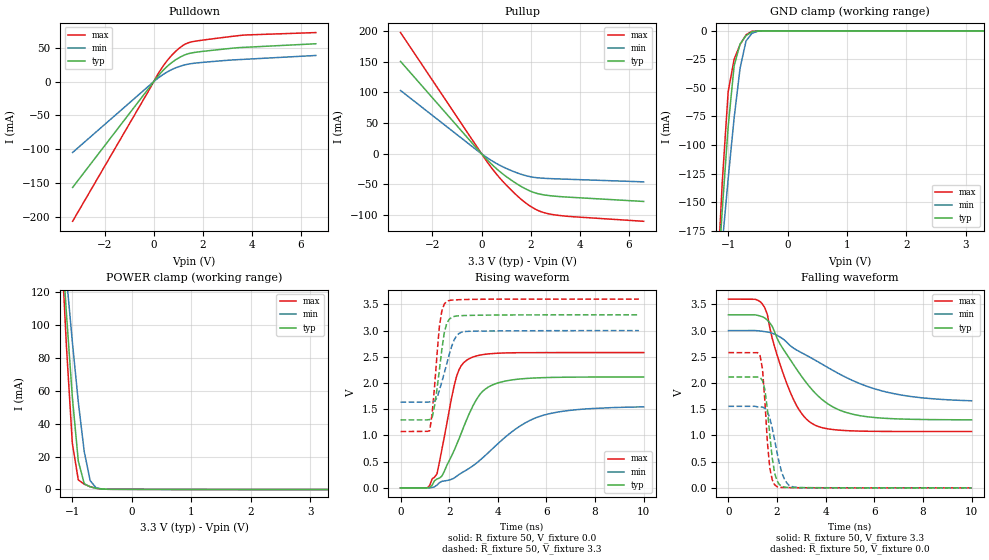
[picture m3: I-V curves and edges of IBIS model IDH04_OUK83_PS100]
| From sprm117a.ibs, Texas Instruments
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[Model]   IDH04_OUK83_PS100
| I/O with pullup
Model_type   I/O
Vinh = 2.00
Vinl = 0.80
Enable   Active-Low
Polarity   Non-Inverting
| signals   A, GZ, Y
Vmeas = 1.5
|   typ   min   max
C_comp   2.866p   2.862p   2.867p
|   typ   min   max
[Temperature Range]   25   -40   125
|   typ   min   max
[Voltage Range]   3.30V   3.00V   3.60V
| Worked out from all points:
|   slope of the pulldown table from 0 to 0.495 V, typ, clamps not added: 23.8 ohm
|   slope of the pullup table from 0 to 0.495 V, typ, clamps not added: 24.4 ohm
|   GND clamp passes 1 mA (typ) near -0.61 V on its own axis
|   POWER clamp passes 1 mA (typ) near -0.64 V on its own axis
|   rising waveform, R_fixture 50, V_fixture 0.0: 20-80 % time 1.24ns typ, 2.52ns min, 660ps max; typ from 0 V to 2.12 V
|   falling waveform, R_fixture 50, V_fixture 3.3: 20-80 % time 1.86ns typ, 3.26ns min, 1.11ns max; typ from 3.3 V to 1.3 V
|   rising waveform, R_fixture 50, V_fixture 3.3: 20-80 % time 341ps typ, 498ps min, 270ps max; typ from 1.3 V to 3.3 V
|   falling waveform, R_fixture 50, V_fixture 0.0: 20-80 % time 302ps typ, 438ps min, 240ps max; typ from 2.12 V to 0 V
[Pulldown]
|   Voltage   I(typ)   I(min)   I(max)
-3.3V     -156.5mA   -104.8mA   -206.6mA
-200mV    -9.762mA   -6.342mA   -13.16mA
200mV     9.308mA    5.91mA     12.77mA
600mV     24.27mA    15.38mA    33.46mA
800mV     30.04mA    19mA       41.54mA
1.1V      36.8mA     23.15mA    51.22mA
1.3V      40.12mA    25.17mA    55.93mA
1.6V      42.95mA    27.12mA    59.33mA
3.5V      50.51mA    32.76mA    68.38mA
6.6V      56.15mA    38.81mA    72.73mA
[GND_clamp]
|   Voltage   I(typ)   I(min)   I(max)
-3.3V     -2.127A    -1.608A    -2.756A
-1.2V     -238.2mA   -246.8mA   -237mA
-1.1V     -157.4mA   -187mA     -133.1mA
-1V       -83.87mA   -129.5mA   -53.38mA
-900mV    -30.72mA   -76.42mA   -25.04mA
-800mV    -11.6mA    -32.84mA   -12.11mA
-700mV    -4.238mA   -8.969mA   -3.556mA
-600mV    -824.9uA   -2.139mA   -405.8uA
-500mV    -75.44uA   -378.5uA   -18.94uA
-400mV    -4.212uA   -46.07uA   -422nA
3.3V      399.7pA    1.987uA    0A
[Pullup]
|   Voltage   I(typ)   I(min)   I(max)
-3.3V     150.6mA    103.2mA    197.6mA
-200mV    9.015mA    6.05mA     12.03mA
300mV     -12.71mA   -8.337mA   -17.25mA
900mV     -34.06mA   -21.94mA   -46.59mA
1.4V      -48.08mA   -30.44mA   -66.63mA
1.8V      -57.38mA   -35.68mA   -80.27mA
2.3V      -65.13mA   -39.22mA   -92.49mA
2.9V      -68.83mA   -40.65mA   -99.12mA
3.7V      -71.1mA    -41.8mA    -102.6mA
6.6V      -77.74mA   -45.8mA    -110.1mA
[POWER_clamp]
|   Voltage   I(typ)   I(min)   I(max)
-3.3V     1.478A     1.119A     1.915A
-1.2V     163.8mA    171.4mA    160.7mA
-1.1V     107.5mA    129.8mA    87.63mA
-1V       56.2mA     89.99mA    28.08mA
-900mV    17.28mA    53.35mA    5.792mA
-800mV    3.493mA    23.02mA    3.135mA
-700mV    1.506mA    5.326mA    1.651mA
-600mV    647.6uA    922.7uA    622.3uA
-500mV    184.9uA    193.5uA    140.8uA
3.3V      -108.3uA   -67.72uA   -162.1uA
[Ramp]
|   I(typ)   I(min)   I(max)
dV/dt_r   1.269/1.231n   0.927/2.521n   1.548/0.657n
dV/dt_f   1.201/1.859n   0.803/3.257n   1.515/1.105n
[Rising Waveform]
R_fixture = 50
V_fixture = 0.0
|  pu_on
|  TIME   V(typ)   V(min)   V(max)
0s        5nV        18nV       5nV
1.1ns     258.5uV    481.5uV    1.899mV
1.5ns     168.2mV    52.31mV    267.3mV
1.7ns     224mV      124.1mV    730mV
2.3ns     816.4mV    218.6mV    2.12V
2.8ns     1.388V     365.6mV    2.458V
3.3ns     1.803V     540.5mV    2.535V
3.7ns     1.946V     710.5mV    2.559V
5.7ns     2.099V     1.359V     2.58V
10ns      2.115V     1.545V     2.58V
[Falling Waveform]
R_fixture = 50
V_fixture = 3.3
V_fixture_min = 3.0
V_fixture_max = 3.6
|  pd_on
|  TIME   V(typ)   V(min)   V(max)
0s        3.3V       3V         3.6V
1.4ns     3.263V     2.987V     3.506V
1.6ns     3.199V     2.973V     3.308V
1.8ns     3.082V     2.95V      2.853V
2.6ns     2.405V     2.692V     1.762V
3.5ns     1.841V     2.453V     1.211V
4.3ns     1.543V     2.239V     1.112V
5.4ns     1.377V     1.99V      1.083V
7.3ns     1.311V     1.756V     1.075V
10ns      1.298V     1.661V     1.075V
[Rising Waveform]
R_fixture = 50
V_fixture = 3.3
V_fixture_min = 3.0
V_fixture_max = 3.6
|  pd_off
|  TIME   V(typ)   V(min)   V(max)
0s        1.297V     1.636V     1.075V
1.2ns     1.303V     1.639V     1.089V
1.3ns     1.335V     1.645V     1.413V
1.4ns     1.569V     1.65V      1.931V
1.6ns     2.255V     1.862V     3.088V
1.7ns     2.642V     2.024V     3.376V
1.9ns     3.135V     2.365V     3.556V
2.2ns     3.27V      2.818V     3.584V
2.6ns     3.287V     2.977V     3.592V
9.8ns     3.3V       3V         3.6V
[Falling Waveform]
R_fixture = 50
V_fixture = 0.0
|  pu_off
|  TIME   V(typ)   V(min)   V(max)
0s        2.115V     1.555V     2.58V
1.3ns     2.109V     1.544V     2.522V
1.4ns     2.045V     1.541V     2.268V
1.5ns     1.872V     1.519V     1.648V
1.7ns     1.01V      1.33V      380.2mV
1.8ns     570.6mV    1.144V     154.5mV
2ns       132.3mV    669.3mV    20.57mV
2.3ns     13.91mV    168.7mV    6.156mV
2.7ns     5.132mV    13.23mV    3.13mV
10ns      3.992uV    80.12uV    415nV
